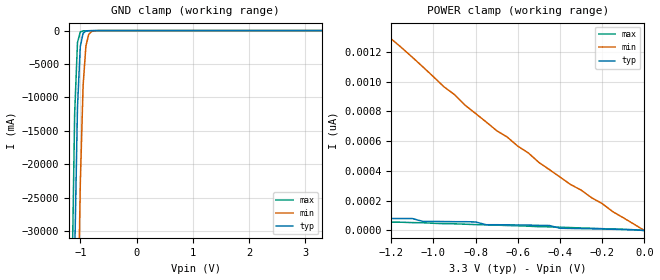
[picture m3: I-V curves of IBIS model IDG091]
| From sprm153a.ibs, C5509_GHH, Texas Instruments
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| Pin_model   IDG091
[Model]   IDG091
 Model_type   Input
 Polarity   Non-Inverting
 Vinl  =  1.08
 Vinh  =  2.10
|Variable   typ   min   max
 C_comp   2.046pF   2.03pF   2.12pF
[Temperature Range]   25   125   -40
[Voltage Range]   3.3   3.0   3.6
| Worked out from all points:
|   GND clamp passes 1 mA (typ) near -0.60 V on its own axis
[GND Clamp]
|Voltage   I(typ)   I(min)   I(max)
-3.3V     -2.127kA   -2.167kA   -2.109kA
-1.15V    -66.48A    -117.1A    -39.31A
-1.1V     -33.84A    -80.11A    -12.46A
-1.05V    -11.54A    -47.82A    -1.806A
-1V       -2.382A    -22.98A    -205mA
-950mV    -392.1mA   -8.238A    -52.03mA
-900mV    -76.18mA   -2.294A    -31.53mA
-850mV    -25.57mA   -572.4mA   -22.71mA
-800mV    -14.01mA   -143.1mA   -15.62mA
-600mV    -1.042mA   -2.237mA   -712.8uA
3.3V      183pA      3.007nA    153.7pA
[POWER Clamp]
|Voltage   I(typ)   I(min)   I(max)
-3.3V     324.6pA    6.189nA    190.5pA
-3.05V    279.3pA    5.317nA    171.9pA
-3V       279.3pA    5.145nA    146.1pA
-2.75V    230.5pA    4.38nA     146.1pA
-2.6V     216.3pA    3.979nA    146.1pA
-2.55V    216.3pA    3.861nA    118.6pA
-1.8V     131.9pA    2.24nA     103.5pA
-1.75V    131.9pA    2.151nA    75.05pA
-1.25V    80.38pA    1.366nA    57.29pA
-700mV    38.64pA    671pA      35.97pA
-350mV    13.77pA    309.1pA    19.54pA
0V        0A         0A         0A
